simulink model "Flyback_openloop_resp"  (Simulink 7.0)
settings: Solver=ode23tb  SolverMode=SingleTasking  StartTime=0.0  StopTime=20e-3  MaxStep=1  RelTol=1e-3
undefined symbols (not defined in the file or in its folder): plecs
libraries: plecslib_extras2 x1

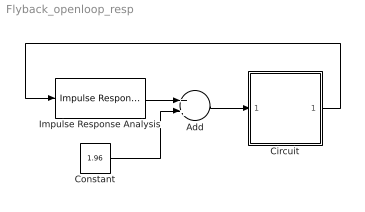
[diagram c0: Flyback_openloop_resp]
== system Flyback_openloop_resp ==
  Add : Sum  OutDataType=sfix(16)  OutScaling=2^-10
  Circuit : Subsystem  LoadFcn=plecs('sl', 200);  InitFcn=plecs('sl', 214);  StartFcn=plecs('sl', 208);  StopFcn=plecs('sl', 209);  mask(PlecsCircuit){PLECSData=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}
      mask prompts: PLECSData "PLECS Data (Do not delete or modify!)"
      mask init:
      | % PLACE CUSTOM INITIALIZATIONS ABOVE
      | % DO NOT REMOVE
      | plecs('sl', 215);
      | % DO NOT REMOVE
  Constant : Constant  Value=1.96  OutDataType=sfix(16)  OutScaling=2^0
  Impulse Response Analysis : plecslib_extras2/Analysis Tools/Impulse Response Analysis  SystemSampleTime=-1  FreqRange=[10 10000]  FreqScale=logarithmic  NPoints=21  Perturbation=1e-3  Compensation=none  TimeSpan=1/50e3  TStart=0  MaxIter=20  Tolerance=1e-6  Display=iteration  HideScopes=on  HiddenStates=error  OutputName=converter  BodePlot=on  JPert=1e-4  NInitCycles=10
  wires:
  Impulse Response Analysis/1 -> Add/1
  Add/1 -> Circuit/1(Vc)
  Constant/1 -> Add/2
  Circuit/1(Vo) -> Impulse Response Analysis/1

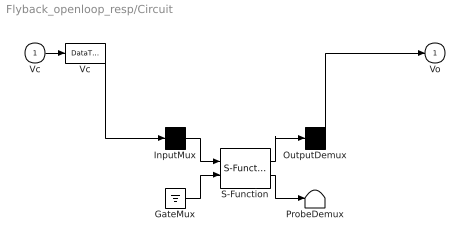
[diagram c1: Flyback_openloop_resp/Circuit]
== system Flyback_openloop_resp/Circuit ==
  Vc : Inport  PortDimensions=1
  " GateMux " : Ground
  " InputMux " : Mux  Inputs=[ 1 ]
  " OutputDemux " : Demux  Outputs=[ 1 ]
  " ProbeDemux " : Terminator
  " S-Function " : S-Function  FunctionName=plecs
  " Vc " : DataTypeConversion
  Vo : Outport  PortDimensions=1
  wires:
  " S-Function "/1 -> " OutputDemux "/1
  " InputMux "/1 -> " S-Function "/1
  " GateMux "/1 -> " S-Function "/2
  " S-Function "/2 -> " ProbeDemux "/1
  Vc/1 -> " Vc "/1
  " Vc "/1 -> " InputMux "/1
  " OutputDemux "/1 -> Vo/1
